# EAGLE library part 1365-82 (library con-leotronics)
DUAL ROW STRAIGHT HEADER 1364 SERIES. 1.27mm x 1.27mm. Without Fixing Post. SMT Source: http://www.leotronics.co.uk/Conexcon/Data%20Sheets/sec.%20A/1364ing.pdf
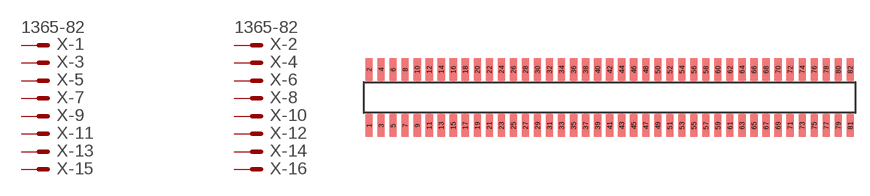
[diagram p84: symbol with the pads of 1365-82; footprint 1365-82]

Designator prefix X; gates -1=MVAL -2=MVAL -3=M -4=M -5=M -6=M -7=M -8=M -9=M -10=M -11=M -12=M -13=M -14=M -15=M -16=M -17=M -18=M -19=M -20=M -21=M -22=M -23=M -24=M -25=M -26=M -27=M -28=M -29=M -30=M -31=M -32=M -33=M -34=M -35=M -36=M -37=M -38=M -39=M -40=M -41=M -42=M -43=M -44=M -45=M -46=M -47=M -48=M -49=M -50=M -51=M -52=M -53=M -54=M -55=M -56=M -57=M -58=M -59=M -60=M -61=M -62=M -63=M -64=M -65=M -66=M -67=M -68=M -69=M -70=M -71=M -72=M -73=M -74=M -75=M -76=M -77=M -78=M -79=M -80=M -81=M -82=M

## 1365-82 (OC_FARNELL: unknown; OC_NEWARK: unknown)  [1365-82]
1  -1:S  pas
2  -2:S  pas
3  -3:S  pas
4  -4:S  pas
5  -5:S  pas
6  -6:S  pas
7  -7:S  pas
8  -8:S  pas
9  -9:S  pas
10  -10:S  pas
11  -11:S  pas
12  -12:S  pas
13  -13:S  pas
14  -14:S  pas
15  -15:S  pas
16  -16:S  pas
17  -17:S  pas
18  -18:S  pas
19  -19:S  pas
20  -20:S  pas
21  -21:S  pas
22  -22:S  pas
23  -23:S  pas
24  -24:S  pas
25  -25:S  pas
26  -26:S  pas
27  -27:S  pas
28  -28:S  pas
29  -29:S  pas
30  -30:S  pas
31  -31:S  pas
32  -32:S  pas
33  -33:S  pas
34  -34:S  pas
35  -35:S  pas
36  -36:S  pas
37  -37:S  pas
38  -38:S  pas
39  -39:S  pas
40  -40:S  pas
41  -41:S  pas
42  -42:S  pas
43  -43:S  pas
44  -44:S  pas
45  -45:S  pas
46  -46:S  pas
47  -47:S  pas
48  -48:S  pas
49  -49:S  pas
50  -50:S  pas
51  -51:S  pas
52  -52:S  pas
53  -53:S  pas
54  -54:S  pas
55  -55:S  pas
56  -56:S  pas
57  -57:S  pas
58  -58:S  pas
59  -59:S  pas
60  -60:S  pas
61  -61:S  pas
62  -62:S  pas
63  -63:S  pas
64  -64:S  pas
65  -65:S  pas
66  -66:S  pas
67  -67:S  pas
68  -68:S  pas
69  -69:S  pas
70  -70:S  pas
71  -71:S  pas
72  -72:S  pas
73  -73:S  pas
74  -74:S  pas
75  -75:S  pas
76  -76:S  pas
77  -77:S  pas
78  -78:S  pas
79  -79:S  pas
80  -80:S  pas
81  -81:S  pas
82  -82:S  pas

## Footprint 1365-82 (pad centres in mm)
DUAL ROW STRAIGHT HEADER 1364 SERIES. 1.27mm x 1.27mm. Without Fixing Post. SMT Source: http://www.leotronics.co.uk/Conexcon/Data%20Sheets/sec.%20A/1364ing.pdf
smd 0.76 x 2.4: 1 -25.4,-2.95; 2 -25.4,2.95; 3 -24.13,-2.95; 4 -24.13,2.95; 5 -22.86,-2.95; 6 -22.86,2.95; 7 -21.59,-2.95; 8 -21.59,2.95; 9 -20.32,-2.95; 10 -20.32,2.95; 11 -19.05,-2.95; 12 -19.05,2.95; 13 -17.78,-2.95; 14 -17.78,2.95; 15 -16.51,-2.95; 16 -16.51,2.95; 17 -15.24,-2.95; 18 -15.24,2.95; 19 -13.97,-2.95; 20 -13.97,2.95; 21 -12.7,-2.95; 22 -12.7,2.95; 23 -11.43,-2.95; 24 -11.43,2.95; 25 -10.16,-2.95; 26 -10.16,2.95; 27 -8.89,-2.95; 28 -8.89,2.95; 29 -7.62,-2.95; 30 -7.62,2.95; 31 -6.35,-2.95; 32 -6.35,2.95; 33 -5.08,-2.95; 34 -5.08,2.95; 35 -3.81,-2.95; 36 -3.81,2.95; 37 -2.54,-2.95; 38 -2.54,2.95; 39 -1.27,-2.95; 40 -1.27,2.95; 41 0,-2.95; 42 0,2.95; 43 1.27,-2.95; 44 1.27,2.95; 45 2.54,-2.95; 46 2.54,2.95; 47 3.81,-2.95; 48 3.81,2.95; 49 5.08,-2.95; 50 5.08,2.95; 51 6.35,-2.95; 52 6.35,2.95; 53 7.62,-2.95; 54 7.62,2.95; 55 8.89,-2.95; 56 8.89,2.95; 57 10.16,-2.95; 58 10.16,2.95; 59 11.43,-2.95; 60 11.43,2.95; 61 12.7,-2.95; 62 12.7,2.95; 63 13.97,-2.95; 64 13.97,2.95; 65 15.24,-2.95; 66 15.24,2.95; 67 16.51,-2.95; 68 16.51,2.95; 69 17.78,-2.95; 70 17.78,2.95; 71 19.05,-2.95; 72 19.05,2.95; 73 20.32,-2.95; 74 20.32,2.95; 75 21.59,-2.95; 76 21.59,2.95; 77 22.86,-2.95; 78 22.86,2.95; 79 24.13,-2.95; 80 24.13,2.95; 81 25.4,-2.95; 82 25.4,2.95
